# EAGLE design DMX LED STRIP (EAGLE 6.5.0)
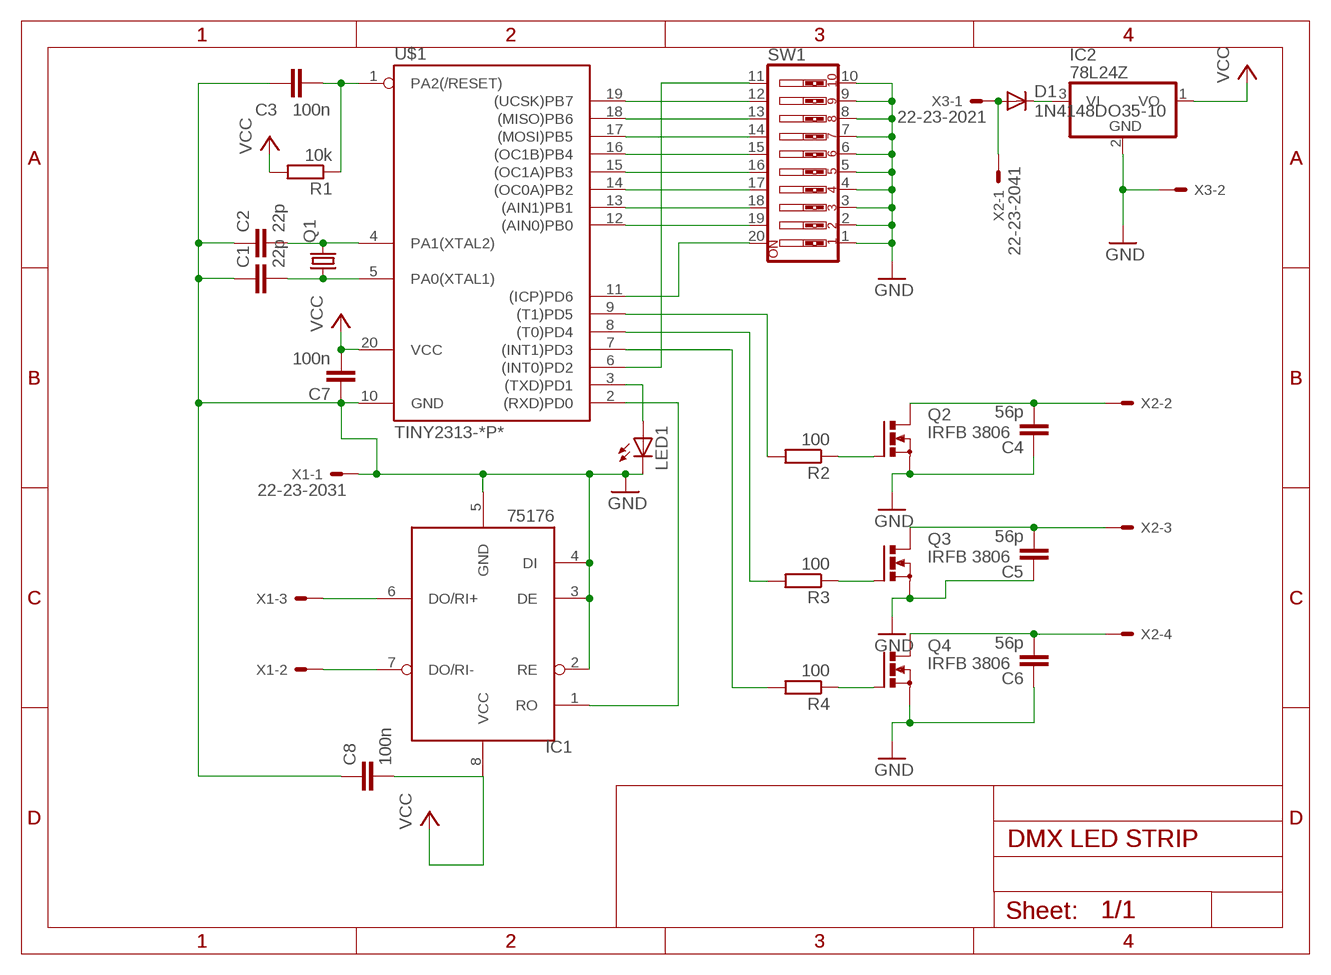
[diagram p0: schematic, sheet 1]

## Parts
C1  22p  C2.5/4  [C2.5-4]
C2  22p  C2.5/4  [C2.5-4]
C3  100n  C2.5/4  [C2.5-4]
C4  56p  C2.5/4  [C2.5-4]
C5  56p  C2.5/4  [C2.5-4]
C6  56p  C2.5/4  [C2.5-4]
C7  100n  C2.5/4  [C2.5-4]
C8  100n  C2.5/4  [C2.5-4]
D1  1N4148DO35-10  [DO35-10]
IC1  75176  [DIL08]
IC2  78L24Z  [TO92]
LED1  LED5MM  [LED5MM]
Q1  CRYSTALHC18U-V  [HC18U-V]
Q2  IRFB 3806  IRF512  [TO220BV]
Q3  IRFB 3806  IRF512  [TO220BV]
Q4  IRFB 3806  IRF512  [TO220BV]
R1  10k  R-EU_0207/10  [0207/10]
R2  100  R-EU_0207/10  [0207/10]
R3  100  R-EU_0207/10  [0207/10]
R4  100  R-EU_0207/10  [0207/10]
SW1  SW_DIP-10  [EDG-10]
U$1  TINY2313-*P*  [DIL20]
X1  22-23-2031  [22-23-2031]
X2  22-23-2041  [22-23-2041]
X3  22-23-2021  [22-23-2021]

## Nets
GND: C1.1 C2.1 C3.1 C4.1 C5.1 C6.1 C7.1 C8.1 IC1.2(RE) IC1.3(DE) IC1.4(DI) IC1.5(GND) IC2.2(GND) LED1.K(C) Q2.S Q3.S Q4.S SW1.1 SW1.2 SW1.3 SW1.4 SW1.5 SW1.6 SW1.7 SW1.8 SW1.9 SW1.10 U$1.10(GND) X1.1 X3.2
N$1: SW1.12 U$1.19((UCSK)PB7)
N$2: SW1.13 U$1.18((MISO)PB6)
N$3: SW1.14 U$1.17((MOSI)PB5)
N$4: SW1.15 U$1.16((OC1B)PB4)
N$5: SW1.16 U$1.15((OC1A)PB3)
N$6: SW1.17 U$1.14((OC0A)PB2)
N$7: SW1.18 U$1.13((AIN1)PB1)
N$8: SW1.19 U$1.12((AIN0)PB0)
N$9: SW1.20 U$1.11((ICP)PD6)
N$10: SW1.11 U$1.6((INT0)PD2)
N$11: IC1.1(RO) U$1.2((RXD)PD0)
N$12: C3.2 R1.1 U$1.1(PA2(/RESET))
N$13: C1.2 Q1.1 U$1.5(PA0(XTAL1))
N$14: IC1.7(DO/RI-) X1.2
N$15: IC1.6(DO/RI+) X1.3
N$16: LED1.A U$1.3((TXD)PD1)
N$17: C2.2 Q1.2 U$1.4(PA1(XTAL2))
N$18: R2.2 U$1.9((T1)PD5)
N$19: R3.2 U$1.8((T0)PD4)
N$20: R4.2 U$1.7((INT1)PD3)
N$21: Q2.G R2.1
N$22: Q3.G R3.1
N$23: Q4.G R4.1
N$24: C4.2 Q2.D X2.2
N$26: C5.2 Q3.D X2.3
N$28: C6.2 Q4.D X2.4
N$29: D1.C IC2.3(VI)
N$30: D1.A X2.1 X3.1
VCC: C7.2 C8.2 IC1.8(VCC) IC2.1(VO) R1.2 U$1.20(VCC)

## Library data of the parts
C1-C8 = capacitor-wima:C: CAPACITOR
D1 = diode:1N4148: DIODE
IC1 = Lutz:75176
IC2 = linear:78*: Positive VOLTAGE REGULATOR Source: http://cache.national.com/ds/LM/LM78L05.pdf http://www.fairchildsemi.com/ds/LM/LM7805.pdf
LED1 = led:LED: LED
Q1 = crystal:CRYSTAL: CRYSTAL; OC_FARNELL: unknown; OC_NEWARK: unknown
Q2-Q4 = transistor-power:IRF512: N-CHANNEL MOS FET
R1-R4 = resistor:R-EU_: RESISTOR, European symbol
SW1 = special:SW_DIP-10: DIP SWITCH
U$1 = avr-6:TINY2313*: Atmel Tiny2313 2K Flash, 128 bytes EEPROM, 128 bytes RAM
X1 = con-molex:22-23-2031: .100" (2.54mm) Center Header - 3 Pin; MF: MOLEX; MPN: 22-23-2031; OC_FARNELL: 1462950; OC_NEWARK: 30C0862
X2 = con-molex:22-23-2041: .100" (2.54mm) Center Header - 4 Pin; MF: MOLEX; MPN: 22-23-2041; OC_FARNELL: 1462920; OC_NEWARK: 38C0355
X3 = con-molex:22-23-2021: .100" (2.54mm) Center Header - 2 Pin; MF: MOLEX; MPN: 22-23-2021; OC_FARNELL: 1462926; OC_NEWARK: 25C3832

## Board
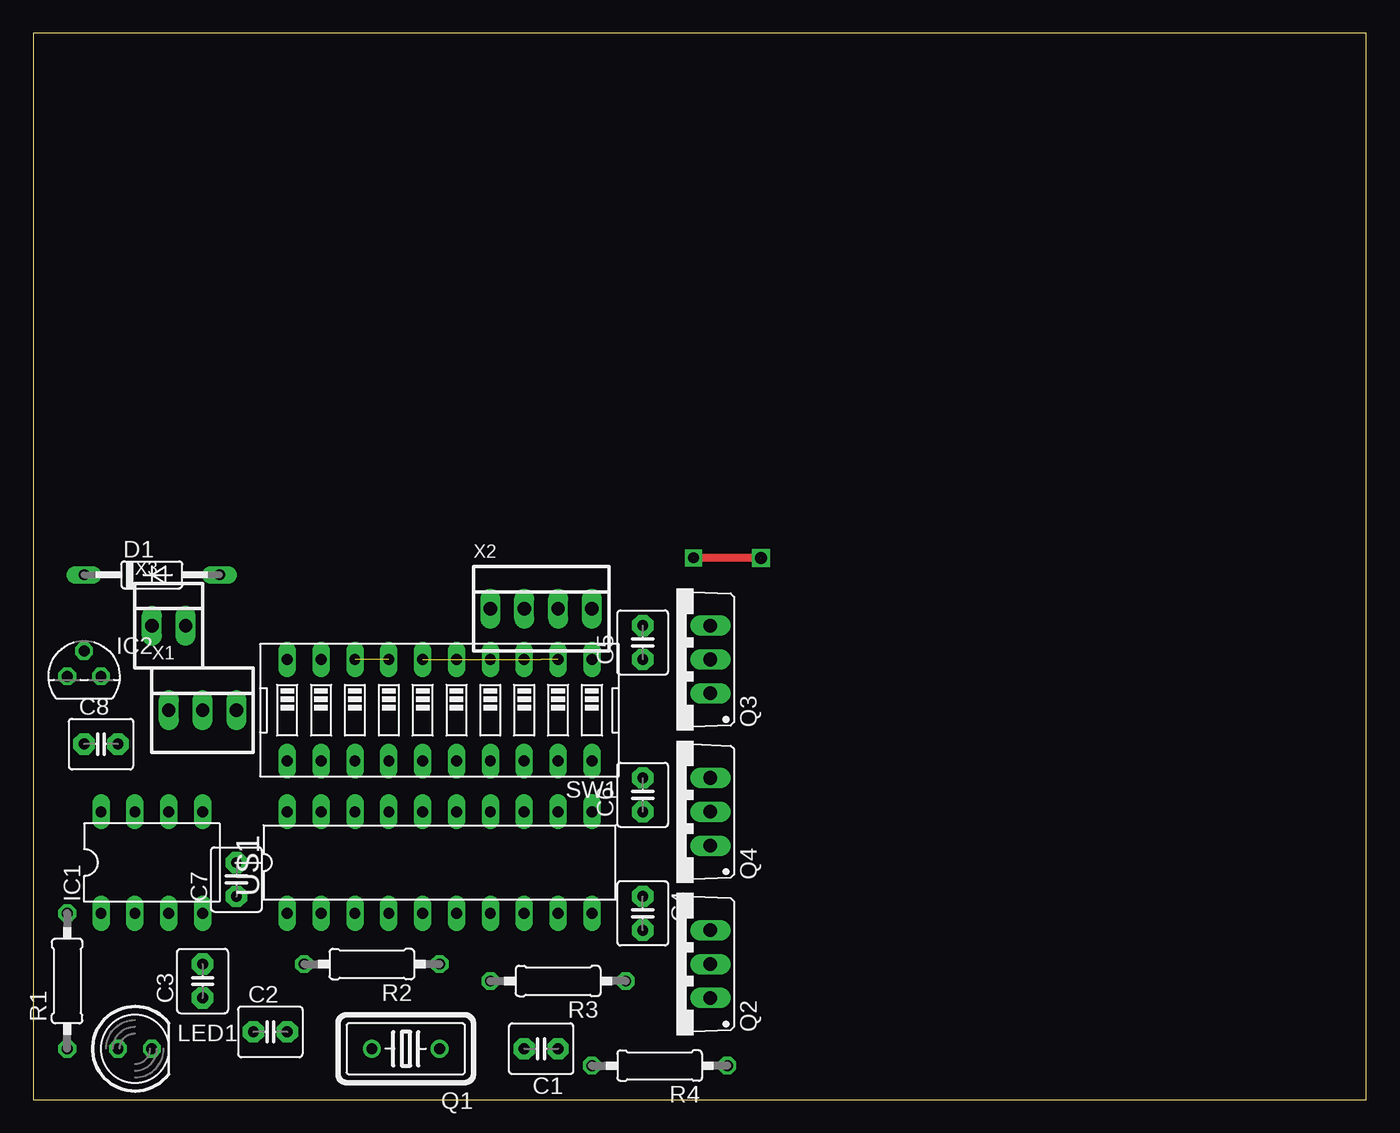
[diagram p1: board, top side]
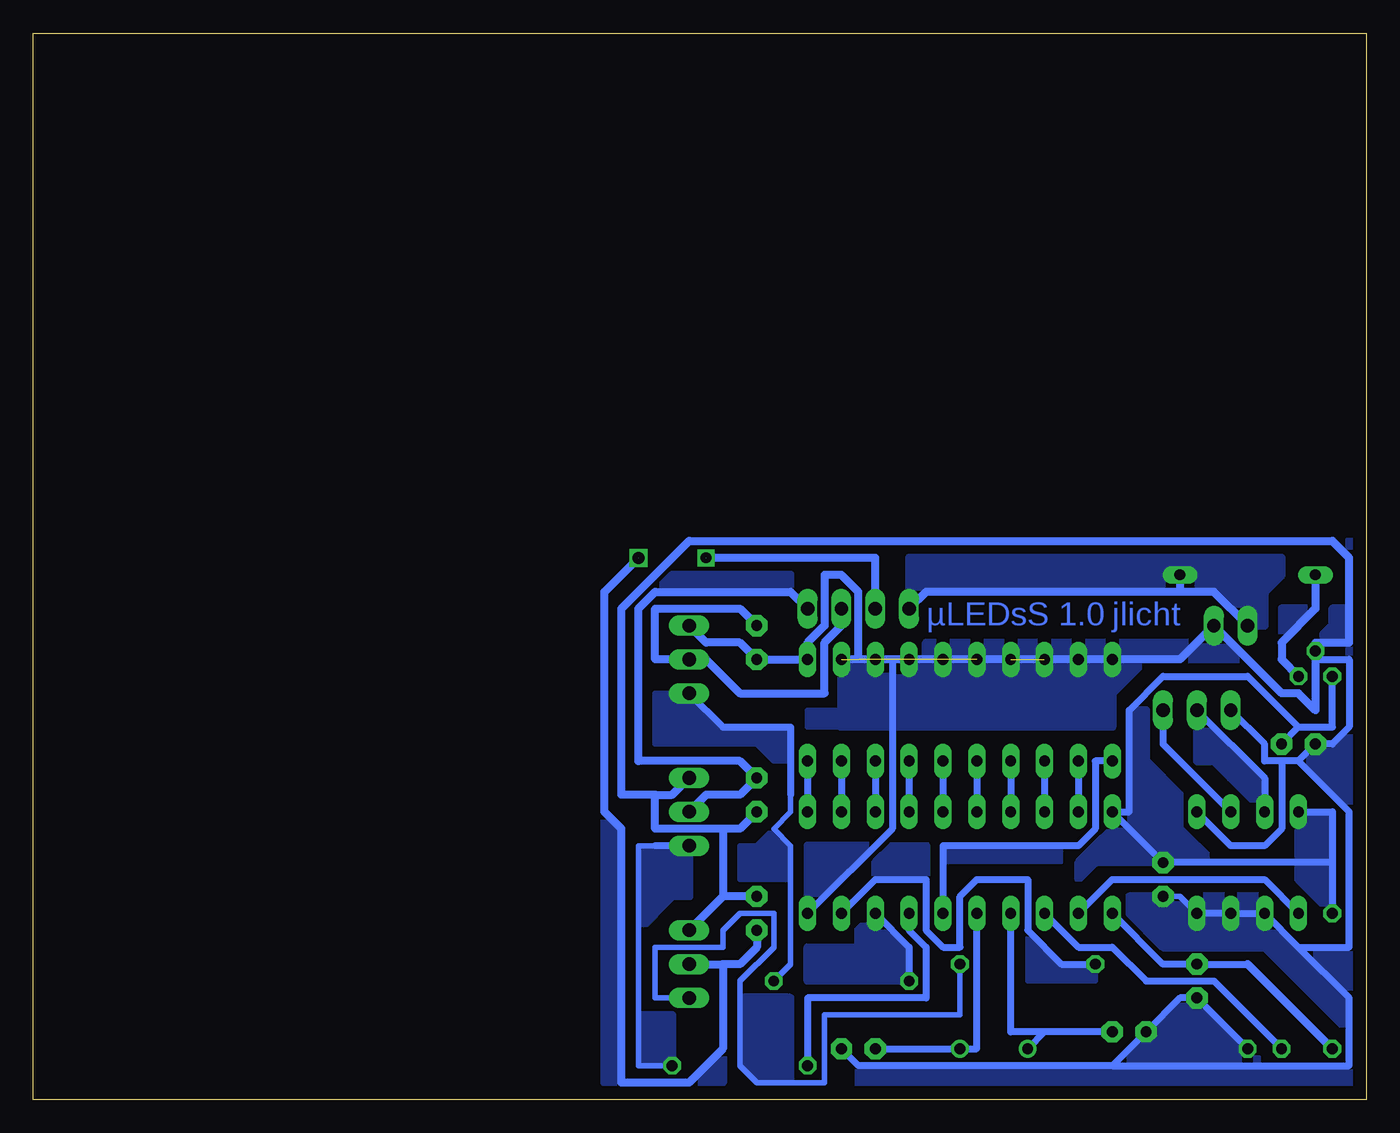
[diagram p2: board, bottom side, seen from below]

Size 100 x 80 mm. Coordinates in mm from the lower left corner, seen from the top.
Outline: 0,0 100,0 100,80 0,80 0,0
Copper layers (1*16): Top 0.035mm / dielectric 1.5mm / Bottom 0.035mm
Design rules "default *": minimum track width 24mil, minimum drill 24mil, track to track 0mil, track to pad 0mil, pad to pad 0mil, via to via 0mil, smd to smd 8mil, copper to edge 40mil, drill to drill 0mil, minimum pad ring 10mil, minimum via ring 8mil, stop-mask expansion 4mil, vias tented up to drill 0mil, thermal gap 10mil

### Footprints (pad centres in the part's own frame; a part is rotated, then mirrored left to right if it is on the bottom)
C2.5-4 = drill 0.813 pad 1.6 octagon: 1 -1.27,0; 2 1.27,0
DO35-10 = drill 0.813 long: A 5.08,0; C -5.08,0
DIL08 = drill 0.813 long: 1 -3.81,-3.81; 2 -1.27,-3.81; 3 1.27,-3.81; 4 3.81,-3.81; 5 3.81,3.81; 6 1.27,3.81; 7 -1.27,3.81; 8 -3.81,3.81
TO92 = drill 0.813 octagon: 1 -1.27,0; 2 0,1.905; 3 1.27,0
LED5MM = drill 0.813 octagon: A -1.27,0; K 1.27,0
HC18U-V = drill 0.813: 1 -2.54,0; 2 2.54,0
TO220BV = drill 1.016 long: D 0,-2.54; G -2.54,-2.54; S 2.54,-2.54
0207/10 = drill 0.813 octagon: 1 -5.08,0; 2 5.08,0
EDG-10 = drill 0.813 long: 1 -11.43,-3.81; 2 -8.89,-3.81; 3 -6.35,-3.81; 4 -3.81,-3.81; 5 -1.27,-3.81; 6 1.27,-3.81; 7 3.81,-3.81; 8 6.35,-3.81; 9 8.89,-3.81; 10 11.43,-3.81; 11 11.43,3.81; 12 8.89,3.81; 13 6.35,3.81; 14 3.81,3.81; 15 1.27,3.81; 16 -1.27,3.81; 17 -3.81,3.81; 18 -6.35,3.81; 19 -8.89,3.81; 20 -11.43,3.81
DIL20 = drill 0.813 long: 1 -11.43,-3.81; 2 -8.89,-3.81; 3 -6.35,-3.81; 4 -3.81,-3.81; 5 -1.27,-3.81; 6 1.27,-3.81; 7 3.81,-3.81; 8 6.35,-3.81; 9 8.89,-3.81; 10 11.43,-3.81; 11 11.43,3.81; 12 8.89,3.81; 13 6.35,3.81; 14 3.81,3.81; 15 1.27,3.81; 16 -1.27,3.81; 17 -3.81,3.81; 18 -6.35,3.81; 19 -8.89,3.81; 20 -11.43,3.81
22-23-2031 = drill 1 long: 1 -2.54,0; 2 0,0; 3 2.54,0
22-23-2041 = drill 1 long: 1 -3.81,0; 2 -1.27,0; 3 1.27,0; 4 3.81,0
22-23-2021 = drill 1 long: 1 -1.27,0; 2 1.27,0

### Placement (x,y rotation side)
C1  38.1,3.81 180 top
C2  17.78,5.08 0 top
C3  12.7,8.89 90 top
C4  45.72,13.97 270 top
C5  45.72,34.29 90 top
C6  45.72,22.86 90 top
C7  15.24,16.51 90 top
C8  5.08,26.67 0 top
D1  8.89,39.37 0 top
IC1  8.89,17.78 0 top
IC2  3.81,31.75 0 top
LED1  7.62,3.81 0 top
Q1  27.94,3.81 180 top
Q2  48.26,10.16 90 top
Q3  48.26,33.02 90 top
Q4  48.26,21.59 90 top
R1  2.54,8.89 90 top
R2  25.4,10.16 180 top
R3  39.37,8.89 180 top
R4  46.99,2.54 180 top
SW1  30.48,29.21 180 top
U$1  30.48,17.78 0 top
X1  12.7,29.21 0 top
X2  38.1,36.83 0 top
X3  10.16,35.56 0 top

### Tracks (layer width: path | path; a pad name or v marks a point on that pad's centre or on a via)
GND  (7 unrouted)
  Bottom 0.406: C7.1 13.97,15.24 IC1.4
  Bottom 0.508: IC1.5 10.16,19.05 7.62,19.05 6.35,20.32 6.35,25.4 | 5.08,25.4 6.35,25.4 | 5.08,25.4 C8.1 2.54,26.67 1.27,27.94 1.27,33.02 3.81,33.02 | X1.1 7.62,26.67 7.62,25.4 6.35,25.4 | IC1.4 IC1.3 IC1.2 5.08,11.43 | LED1.K C3.1 13.97,7.62 C2.1 19.05,2.54 | C1.1 38.1,2.54 19.05,2.54 | 5.08,11.43 1.27,7.62 1.27,2.54 19.05,2.54 | 5.08,25.4 1.27,21.59 1.27,11.43 5.08,11.43 | U$1.10 35.56,20.32 35.56,33.02
  Bottom 0.61: Q3.S 49.53,34.29 46.99,34.29 C5.1 SW1.1 41.91,34.29 40.64,35.56 40.64,39.37 39.37,39.37 38.1,38.1 38.1,33.02 | 48.26,15.24 Q2.S | C4.1 48.26,15.24 | Q4.S 52.07,22.86 53.34,22.86 | 53.34,22.86 53.34,20.32 48.26,20.32 | 48.26,20.32 46.99,20.32 C6.1 | 48.26,20.32 48.26,15.24 | 53.34,22.86 55.88,22.86 55.88,36.83 50.8,41.91 2.54,41.91 1.27,40.64 1.27,34.29 3.81,34.29 IC2.2 3.81,33.02 3.81,29.21 5.08,30.48 6.35,30.48 X3.2 13.97,33.02 SW1.10 SW1.9 SW1.8 SW1.2
N$1
  Bottom 0.508: SW1.12 U$1.19
N$2
  Bottom 0.508: SW1.13 U$1.18
N$3
  Bottom 0.508: SW1.14 U$1.17
N$4
  Bottom 0.508: SW1.15 U$1.16
N$5
  Bottom 0.508: SW1.16 U$1.15
N$6
  Bottom 0.508: SW1.17 U$1.14
N$7
  Bottom 0.508: SW1.18 U$1.13
N$8
  Bottom 0.508: SW1.19 U$1.12
N$9
  Bottom 0.508: SW1.20 U$1.11
N$10
  Bottom 0.508: U$1.6 31.75,19.05 21.59,19.05 20.32,20.32 20.32,25.4 SW1.11
N$11
  Bottom 0.508: IC1.1 7.62,16.51 19.05,16.51 U$1.2
N$12
  Bottom 0.508: 8.89,10.16 C3.2 15.24,10.16 U$1.1
  Bottom 0.61: 8.89,10.16 R1.1
N$13
  Bottom 0.508: C1.2 Q1.1 29.21,3.81 U$1.5
N$14
  Bottom 0.508: IC1.7 7.62,24.13 X1.2
N$15
  Bottom 0.508: IC1.6 15.24,26.67 X1.3
N$16
  Bottom 0.508: LED1.A 11.43,8.89 16.51,8.89 19.05,11.43 21.59,11.43 U$1.3
N$17
  Bottom 0.508: 24.13,5.08 Q1.2 | C2.2 24.13,5.08 | U$1.4 26.67,5.08 24.13,5.08
N$18
  Bottom 0.508: R2.2 22.86,10.16 25.4,12.7 25.4,16.51 29.21,16.51 30.48,15.24 30.48,11.43 31.75,11.43 33.02,12.7 33.02,16.51 36.83,16.51 U$1.9
N$19
  Bottom 0.508: R3.2 34.29,11.43 U$1.8
N$20
  Bottom 0.508: R4.2 41.91,7.62 33.02,7.62 33.02,11.43 34.29,12.7 U$1.7
N$21
  Bottom 0.406: R2.1 30.48,6.35 40.64,6.35 40.64,1.27 45.72,1.27 46.99,2.54 46.99,8.89 44.45,11.43 44.45,13.97 46.99,13.97 48.26,12.7 48.26,11.43 53.34,11.43 53.34,7.62 Q2.G
N$22
  Bottom 0.406: R3.1 43.18,10.16 43.18,19.05 44.45,20.32 43.18,21.59 43.18,22.86
  Bottom 0.508: 43.18,22.86 43.18,27.94 48.26,27.94 Q3.G
N$23
  Bottom 0.406: 53.34,19.05 54.61,19.05 54.61,2.54 R4.1
  Bottom 0.508: Q4.G 53.34,19.05
N$24  (2 unrouted)
  Top 0.61: 54.61,40.64 49.53,40.64
  Bottom 0.61: Q2.D 48.26,10.16 | X2.2 36.83,40.64 49.53,40.64 | C4.2 45.72,11.43 46.99,10.16 48.26,10.16 | 48.26,10.16 48.26,3.81 50.8,1.27 55.88,1.27 55.88,20.32 57.15,21.59 57.15,38.1 54.61,40.64
N$25  (via drill 0.8 pad 1.27)
  other vias: 49.53,40.64
N$26
  Bottom 0.61: X2.3 39.37,35.56 40.64,34.29 40.64,30.48 46.99,30.48 49.53,33.02 Q3.D 53.34,33.02 53.34,36.83 46.99,36.83 C5.2
N$27
  pour Bottom: 16.51,33.02 19.05,30.48 19.05,27.94 39.37,27.94 39.37,33.02
N$28
  Bottom 0.61: X2.4 43.18,38.1 53.34,38.1 54.61,36.83 54.61,25.4 46.99,25.4 C6.2 46.99,22.86 49.53,22.86 Q4.D
N$29
  Bottom 0.61: D1.C 3.81,36.83 6.35,34.29 6.35,33.02 IC2.3
N$30
  Bottom 0.61: X3.1 11.43,38.1 13.97,38.1 | 13.97,38.1 33.02,38.1 X2.1 | D1.A 13.97,38.1
N$31
  pour Bottom: 12.7,38.1 11.43,38.1 8.89,35.56 7.62,35.56 7.62,38.1 6.35,39.37 6.35,40.64 34.29,40.64 34.29,36.83 33.02,38.1
N$32
  pour Bottom: 38.1,2.54 38.1,1.27 38.1,0 0,0 0,41.91 1.27,41.91 1.27,27.94 2.54,26.67 3.81,26.67 5.08,25.4 1.27,21.59 1.27,11.43 5.08,11.43 1.27,7.62 1.27,2.54 7.62,2.54 8.89,3.81 12.7,7.62 13.97,7.62 19.05,2.54
N$33
  pour Bottom: 11.43,17.78 13.97,20.32 13.97,22.86 16.51,25.4 16.51,29.21 17.78,29.21 17.78,21.59 19.05,21.59 15.24,17.78
N$34
  pour Bottom: 1.27,7.62 7.62,13.97 7.62,15.24 17.78,15.24 17.78,13.97 15.24,11.43 7.62,11.43 1.27,5.08
N$35
  pour Bottom: 15.24,17.78 20.32,17.78 21.59,16.51 21.59,17.78 17.78,21.59 17.78,20.32
N$36
  pour Bottom: 43.18,1.27 43.18,7.62 46.99,7.62 46.99,2.54 45.72,1.27
N$37
  pour Bottom: 36.83,13.97 34.29,11.43 34.29,8.89 41.91,8.89 41.91,11.43 38.1,11.43 38.1,12.7
N$38
  pour Bottom: 5.08,21.59 5.08,16.51 2.54,13.97 2.54,21.59
N$39
  pour Bottom: 12.7,29.21 12.7,25.4 11.43,25.4 10.16,24.13 7.62,21.59 7.62,24.13
N$40
  pour Bottom: 50.8,19.05 50.8,15.24 52.07,15.24 54.61,12.7 54.61,19.05
N$41
  pour Bottom: 52.07,2.54 54.61,2.54 54.61,6.35 52.07,6.35
N$42
  pour Bottom: 36.83,19.05 41.91,19.05 41.91,13.97
N$43
  pour Bottom: 43.18,16.51 46.99,16.51 46.99,19.05 45.72,19.05 44.45,20.32 43.18,19.05
N$44
  pour Bottom: 43.18,38.1 43.18,39.37 52.07,39.37 53.34,38.1
N$45
  pour Bottom: 43.18,25.4 44.45,25.4 45.72,26.67 53.34,26.67 53.34,30.48 50.8,30.48 48.26,27.94 43.18,27.94
N$46  (via drill 0.9 pad 1.27)
  other vias: 54.61,40.64
N$47
  pour Bottom: 1.27,36.83 2.54,36.83 2.54,35.56 3.81,34.29 1.27,34.29
N$48
  pour Bottom: 55.88,1.27 57.15,1.27 57.15,21.59 55.88,20.32
N$49
  pour Bottom: 48.26,3.81 48.26,1.27 50.8,1.27
N$50
  pour Bottom: 33.02,34.29 12.7,34.29 13.97,33.02 33.02,33.02
N$51
  pour Bottom: 10.16,33.02 13.97,33.02 11.43,35.56 8.89,33.02
N$52
  pour Bottom: 35.56,19.05 33.02,19.05 33.02,16.51 36.83,16.51 36.83,17.78
N$53
  pour Bottom: 31.75,17.78 22.86,17.78 22.86,19.05 31.75,19.05
N$54
  pour Bottom: 20.32,10.16 20.32,8.89 25.4,8.89 25.4,12.7 22.86,10.16
N$55
  pour Bottom: 39.37,27.94 41.91,27.94 41.91,29.21 39.37,29.21
N$56
  pour Bottom: 3.81,36.83 6.35,36.83 6.35,34.29
VCC
  Bottom 0.508: IC2.1 2.54,27.94 5.08,27.94 | C8.2 5.08,27.94 | 2.54,17.78 2.54,21.59 IC1.8 | 2.54,17.78 R1.2 | 2.54,17.78 C7.2 U$1.20 17.78,21.59 17.78,29.21 15.24,31.75 8.89,31.75 5.08,27.94

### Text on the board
Bottom: jlicht | µLEDsS 1.0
